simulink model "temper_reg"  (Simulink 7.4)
settings: Solver=ode45  StartTime=0.0  StopTime=24  MaxStep=0.1  RelTol=1e-3  AbsTol=1e-3
undefined symbols (not defined in the file or in its folder): sigbuilder_block

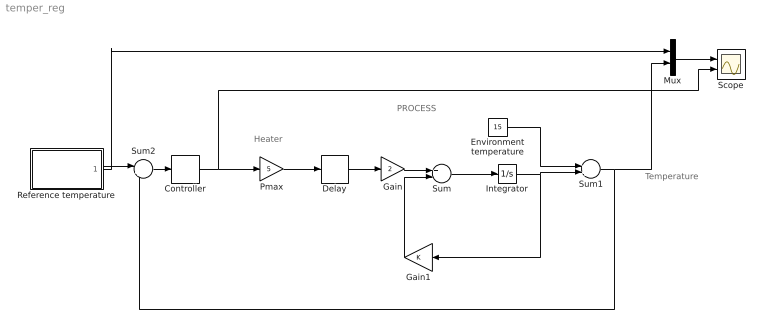
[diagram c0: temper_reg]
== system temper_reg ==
  note: PROCESS
  note: Heater
  note: Temperature
  Controller : Relay  OnSwitchValue=0.5  OffSwitchValue=-0.5  OutDataType=sfix(16)  OutScaling=2^0
  Delay : TransportDelay  DelayTime=0.1
  Environment temperature : Constant  Value=15  OutDataType=sfix(16)  OutScaling=2^0
  Gain : Gain  Gain=2  ParameterDataType=sfix(16)  ParameterScaling=2^0  OutDataType=sfix(16)  OutScaling=2^0
  Gain1 : Gain  ParameterDataType=sfix(16)  ParameterScaling=2^0  OutDataType=sfix(16)  OutScaling=2^0
  Integrator : Integrator  InitialCondition=1
  Mux : Mux  Inputs=2
  Pmax : Gain  Gain=5  ParameterDataType=sfix(16)  ParameterScaling=2^0  OutDataType=sfix(16)  OutScaling=2^0
  Reference temperature : Subsystem  Tag=STV Subsys  LoadFcn=sigbuilder_block('load');  StartFcn=sigbuilder_block('start');  StopFcn=sigbuilder_block('stop');  ClipboardFcn=sigbuilder_block('clipboard');
  Scope : Scope  NumInputPorts=2
  Sum : Sum  Inputs=+-  OutDataType=sfix(16)  OutScaling=2^0
  Sum1 : Sum  OutDataType=sfix(16)  OutScaling=2^0
  Sum2 : Sum  Inputs=|+-  OutDataType=sfix(16)  OutScaling=2^0
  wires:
  Gain/1 -> Sum/1
  Sum/1 -> Integrator/1
  Gain1/1 -> Sum/2
  Integrator/1 -> Gain1/1, Sum1/2
  Environment temperature/1 -> Sum1/1
  Reference temperature/1(Signal 1) -> Sum2/1, Mux/1
  Sum1/1 -> Sum2/2, Mux/2
  Sum2/1 -> Controller/1
  Delay/1 -> Gain/1
  Controller/1 -> Pmax/1, Scope/2
  Pmax/1 -> Delay/1
  Mux/1 -> Scope/1

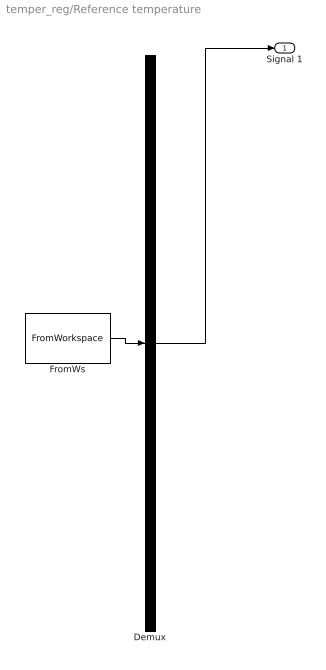
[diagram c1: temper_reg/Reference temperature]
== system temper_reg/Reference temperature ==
  Demux : Demux  Tag=STV Demux  Outputs=1
  FromWs : FromWorkspace  Tag=STV FromWs  VariableName=tuvar  SampleTime=0  SigBuilderData=DataTag0  VnvData=DataTag1
  Signal 1 : Outport  Tag=STV Outport  OutDataType=sfix(16)  OutScaling=2^0
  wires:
  Demux/1 -> Signal 1/1
  FromWs/1 -> Demux/1
